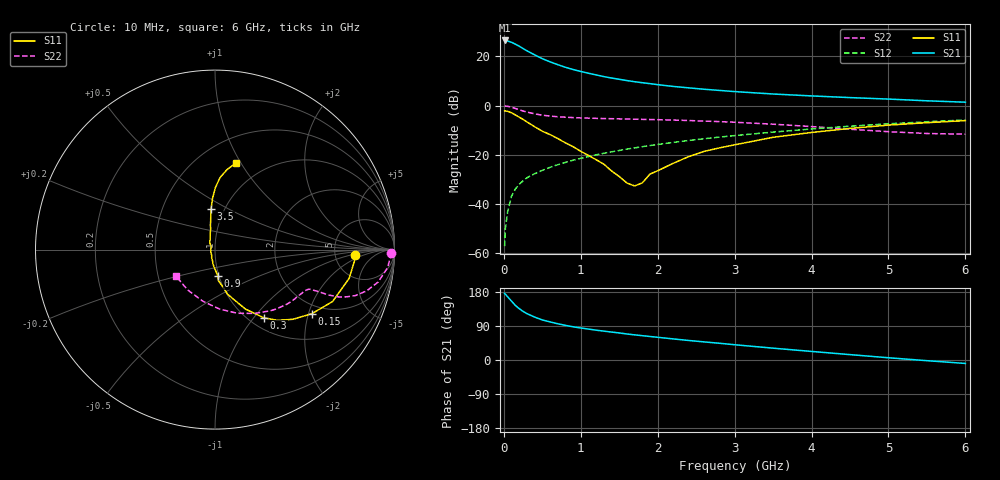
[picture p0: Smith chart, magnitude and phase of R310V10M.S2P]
! SIEMENS Small Signal Semiconductors
! BFR181
! Si NPN RF Bipolar Junction Transistor in SOT23
! VCE = 10 V  IC = 10 mA
! Common Emitter S-Parameters:  May  1996
# GHz  S  MA  R  50
!  f  S11  S21  S12  S22
! GHz  MAG  ANG  MAG  ANG  MAG  ANG  MAG  ANG
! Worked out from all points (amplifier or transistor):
!   36 points, 10 MHz to 6 GHz, reference 50 ohm
!   highest |S21| = 26.5 dB at 10 MHz (marker M1)
!   |S21| within 3 dB of that: start of sweep to 235.4 MHz
!   unconditionally stable (mu >= 1): 894.6 MHz to 2.896 GHz
!   at 250 MHz: K = 0.58, MSG = 26.9 dB, |S12| = -30.5 dB
!   at 1.4 GHz: K = 1.05, MAG = 13.7 dB, |S12| = -18.8 dB
!   at 6 GHz: K = 0.87, MSG = 3.6 dB, |S12| = -5.8 dB
!   S11 on the Smith chart (normalised r, x): 10 MHz: 7.88, -1.32; 150 MHz: 1.71, -2.10; 300 MHz: 1.16, -1.13; 900 MHz: 0.99, -0.29; 3.5 GHz: 0.87, +0.41; 6 GHz: 0.74, +0.95
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0.01  0.7802 -2.4  21.05 175.8  0.0014 83.6  0.9817 -1.0
0.02  0.7798 -4.6  20.67 173.6  0.0032 86.1  0.9778 -2.4
0.05  0.7644 -12.1  20.52 166.7  0.0071 81.6  0.9672 -5.9
0.1  0.7163 -23.8  19.32 155.3  0.0145 78.4  0.9273 -11.2
0.15  0.6471 -33.5  17.67 144.0  0.0203 73.6  0.8761 -15.2
0.2  0.5817 -41.9  16.11 135.5  0.0253 71.8  0.8239 -18.1
0.25  0.5252 -48.6  14.43 128.2  0.0298 69.6  0.7773 -19.8
0.3  0.4673 -54.4  12.98 122.4  0.0343 68.9  0.7406 -20.9
0.4  0.3732 -62.8  10.75 113.3  0.0414 68.3  0.6805 -21.8
0.5  0.3021 -68.8  8.981 105.7  0.0485 68.7  0.6393 -22.0
0.6  0.2587 -74.2  7.75 100.5  0.0559 68.6  0.6143 -22.2
0.7  0.2153 -77.7  6.799 95.7  0.063 68.9  0.5946 -22.4
0.9  0.1467 -84.1  5.416 87.6  0.0779 69.1  0.5715 -22.7
1.1  0.0973 -93.1  4.548 81.6  0.0925 69.1  0.5567 -23.9
1.4  0.0472 -113.7  3.633 73.7  0.1151 68.5  0.5428 -26.4
1.7  0.0234 170.2  3.058 66.3  0.1386 67.1  0.5305 -29.2
2.2  0.0672 113.5  2.456 55.7  0.1789 64.0  0.5093 -35.5
2.8  0.1383 100.6  2.036 44.2  0.2293 59.6  0.4741 -44.4
3.5  0.2276 95.5  1.721 31.2  0.2901 53.3  0.4197 -57.9
4.5  0.3446 89.7  1.455 14.2  0.3822 42.8  0.3316 -85.8
5.5  0.4503 81.5  1.253 -1.8  0.4704 30.7  0.2716 -123.9
6  0.496 76.5  1.174 -9.1  0.5114 24.0  0.2632 -145.7
